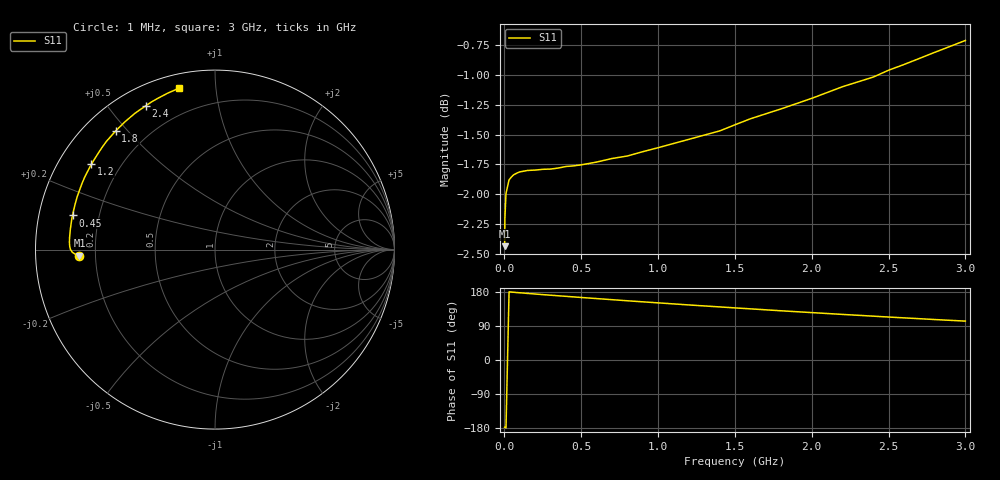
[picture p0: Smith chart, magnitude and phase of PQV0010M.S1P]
! SIEMENS Small Signal Semiconductors
! BAR64-04
! Si PIN Diode in SOT23 (2 diodes in series, pin 3 open)
! IF = 10 mA
! S-Parameters:  July  1992
# GHz  S  MA  R  50
!  f  S11
! GHz  MAG  ANG
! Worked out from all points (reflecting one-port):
!   33 points, 1 MHz to 3 GHz, reference 50 ohm
!   lowest |S11| = -2.4 dB at 1 MHz (marker M1), VSWR 7.19, Z = 6.96 - j1.07 ohm
!   phase of S11 starts at -178 deg and turns -80 deg over the sweep
!   S11 on the Smith chart (normalised r, x): 1 MHz: 0.14, -0.02; 450 MHz: 0.10, +0.12; 1.2 GHz: 0.10, +0.31; 1.8 GHz: 0.09, +0.46; 2.4 GHz: 0.08, +0.63; 3 GHz: 0.07, +0.80
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0.001  0.7557 -177.5
0.003  0.7764 -178.0
0.01  0.795 -178.9
0.03  0.8055 179.9
0.05  0.8083 179.1
0.06  0.8094 178.8
0.08  0.8107 178.0
0.1  0.8117 177.4
0.15  0.8128 175.7
0.25  0.8137 172.5
0.4  0.8159 168.0
0.45  0.8164 166.5
0.6  0.8194 162.1
0.7  0.8222 159.2
0.8  0.8242 156.3
0.9  0.8276 153.5
1  0.8308 150.8
1.2  0.8375 145.3
1.5  0.8493 137.5
1.6  0.8542 135.0
1.8  0.8624 129.9
2  0.8712 125.1
2.2  0.881 120.3
2.4  0.8892 115.7
2.5  0.8951 113.4
2.6  0.9 111.2
2.8  0.9106 106.8
3  0.9211 102.6
